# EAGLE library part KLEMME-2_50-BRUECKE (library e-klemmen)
Klemme 50-pol. mit Brückenhinweis
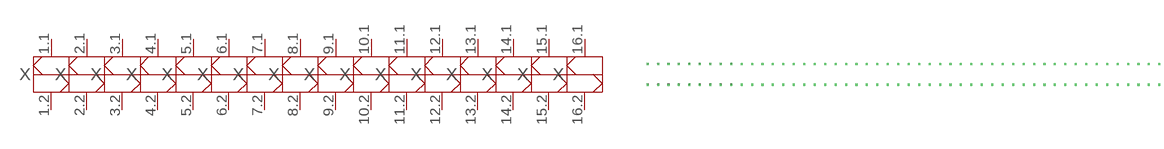
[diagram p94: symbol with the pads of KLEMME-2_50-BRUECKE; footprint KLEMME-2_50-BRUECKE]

Designator prefix X; gates 1=KLEMME-2_1-BRUECKE 2=KLEMME-2_2-BRUECKE 3=KLEMME-2_3-BRUECKE 4=KLEMME-2_4-BRUECKE 5=KLEMME-2_5-BRUECKE 6=KLEMME-2_6-BRUECKE 7=KLEMME-2_7-BRUECKE 8=KLEMME-2_8-BRUECKE 9=KLEMME-2_9-BRUECKE 10=KLEMME-2_10-BRUECKE 11=KLEMME-2_11-BRUECKE 12=KLEMME-2_12-BRUECKE 13=KLEMME-2_13-BRUECKE 14=KLEMME-2_14-BRUECKE 15=KLEMME-2_15-BRUECKE 16=KLEMME-2_16-BRUECKE 17=KLEMME-2_17-BRUECKE 18=KLEMME-2_18-BRUECKE 19=KLEMME-2_19-BRUECKE 20=KLEMME-2_20-BRUECKE 21=KLEMME-2_21-BRUECKE 22=KLEMME-2_22-BRUECKE 23=KLEMME-2_23-BRUECKE 24=KLEMME-2_24-BRUECKE 25=KLEMME-2_25-BRUECKE 26=KLEMME-2_26-BRUECKE 27=KLEMME-2_27-BRUECKE 28=KLEMME-2_28-BRUECKE 29=KLEMME-2_29-BRUECKE 30=KLEMME-2_30-BRUECKE 31=KLEMME-2_31-BRUECKE 32=KLEMME-2_32-BRUECKE 33=KLEMME-2_33-BRUECKE 34=KLEMME-2_34-BRUECKE 35=KLEMME-2_35-BRUECKE 36=KLEMME-2_36-BRUECKE 37=KLEMME-2_37-BRUECKE 38=KLEMME-2_38-BRUECKE 39=KLEMME-2_39-BRUECKE 40=KLEMME-2_40-BRUECKE 41=KLEMME-2_41-BRUECKE 42=KLEMME-2_42-BRUECKE 43=KLEMME-2_43-BRUECKE 44=KLEMME-2_44-BRUECKE 45=KLEMME-2_45-BRUECKE 46=KLEMME-2_46-BRUECKE 47=KLEMME-2_47-BRUECKE 48=KLEMME-2_48-BRUECKE 49=KLEMME-2_49-BRUECKE 50=KLEMME-2_50-BRUECKE

## KLEMME-2_50-BRUECKE  [KLEMME-2_50-BRUECKE]
1.1  1:1  pas
1.2  1:2  pas
2.1  2:1  pas
2.2  2:2  pas
3.1  3:1  pas
3.2  3:2  pas
4.1  4:1  pas
4.2  4:2  pas
5.1  5:1  pas
5.2  5:2  pas
6.1  6:1  pas
6.2  6:2  pas
7.1  7:1  pas
7.2  7:2  pas
8.1  8:1  pas
8.2  8:2  pas
9.1  9:1  pas
9.2  9:2  pas
10.1  10:1  pas
10.2  10:2  pas
11.1  11:1  pas
11.2  11:2  pas
12.1  12:1  pas
12.2  12:2  pas
13.1  13:1  pas
13.2  13:2  pas
14.1  14:1  pas
14.2  14:2  pas
15.1  15:1  pas
15.2  15:2  pas
16.1  16:1  pas
16.2  16:2  pas
17.1  17:1  pas
17.2  17:2  pas
18.1  18:1  pas
18.2  18:2  pas
19.1  19:1  pas
19.2  19:2  pas
20.1  20:1  pas
20.2  20:2  pas
21.1  21:1  pas
21.2  21:2  pas
22.1  22:1  pas
22.2  22:2  pas
23.1  23:1  pas
23.2  23:2  pas
24.1  24:1  pas
24.2  24:2  pas
25.1  25:1  pas
25.2  25:2  pas
26.1  26:1  pas
26.2  26:2  pas
27.1  27:1  pas
27.2  27:2  pas
28.1  28:1  pas
28.2  28:2  pas
29.1  29:1  pas
29.2  29:2  pas
30.1  30:1  pas
30.2  30:2  pas
31.1  31:1  pas
31.2  31:2  pas
32.1  32:1  pas
32.2  32:2  pas
33.1  33:1  pas
33.2  33:2  pas
34.1  34:1  pas
34.2  34:2  pas
35.1  35:1  pas
35.2  35:2  pas
36.1  36:1  pas
36.2  36:2  pas
37.1  37:1  pas
37.2  37:2  pas
38.1  38:1  pas
38.2  38:2  pas
39.1  39:1  pas
39.2  39:2  pas
40.1  40:1  pas
40.2  40:2  pas
41.1  41:1  pas
41.2  41:2  pas
42.1  42:1  pas
42.2  42:2  pas
43.1  43:1  pas
43.2  43:2  pas
44.1  44:1  pas
44.2  44:2  pas
45.1  45:1  pas
45.2  45:2  pas
46.1  46:1  pas
46.2  46:2  pas
47.1  47:1  pas
47.2  47:2  pas
48.1  48:1  pas
48.2  48:2  pas
49.1  49:1  pas
49.2  49:2  pas
50.1  50:1  pas
50.2  50:2  pas

## Footprint KLEMME-2_50-BRUECKE (pad centres in mm)
Dummy
drill 0.5 pad 1 square: 1.1 0,-2.54; 1.2 0,-12.7; 2.1 5.08,-2.54; 2.2 5.08,-12.7; 3.1 10.16,-2.54; 3.2 10.16,-12.7; 4.1 15.24,-2.54; 4.2 15.24,-12.7; 5.1 20.32,-2.54; 5.2 20.32,-12.7; 6.1 25.4,-2.54; 6.2 25.4,-12.7; 7.1 30.48,-2.54; 7.2 30.48,-12.7; 8.1 35.56,-2.54; 8.2 35.56,-12.7; 9.1 40.64,-2.54; 9.2 40.64,-12.7; 10.1 45.72,-2.54; 10.2 45.72,-12.7; 11.1 50.8,-2.54; 11.2 50.8,-12.7; 12.1 55.88,-2.54; 12.2 55.88,-12.7; 13.1 60.96,-2.54; 13.2 60.96,-12.7; 14.1 66.04,-2.54; 14.2 66.04,-12.7; 15.1 71.12,-2.54; 15.2 71.12,-12.7; 16.1 76.2,-2.54; 16.2 76.2,-12.7; 17.1 81.28,-2.54; 17.2 81.28,-12.7; 18.1 86.36,-2.54; 18.2 86.36,-12.7; 19.1 91.44,-2.54; 19.2 91.44,-12.7; 20.1 96.52,-2.54; 20.2 96.52,-12.7; 21.1 101.6,-2.54; 21.2 101.6,-12.7; 22.1 106.68,-2.54; 22.2 106.68,-12.7; 23.1 111.76,-2.54; 23.2 111.76,-12.7; 24.1 116.84,-2.54; 24.2 116.84,-12.7; 25.1 121.92,-2.54; 25.2 121.92,-12.7; 26.1 127,-2.54; 26.2 127,-12.7; 27.1 132.08,-2.54; 27.2 132.08,-12.7; 28.1 137.16,-2.54; 28.2 137.16,-12.7; 29.1 142.24,-2.54; 29.2 142.24,-12.7; 30.1 147.32,-2.54; 30.2 147.32,-12.7; 31.1 152.4,-2.54; 31.2 152.4,-12.7; 32.1 157.48,-2.54; 32.2 157.48,-12.7; 33.1 162.56,-2.54; 33.2 162.56,-12.7; 34.1 167.64,-2.54; 34.2 167.64,-12.7; 35.1 172.72,-2.54; 35.2 172.72,-12.7; 36.1 177.8,-2.54; 36.2 177.8,-12.7; 37.1 182.88,-2.54; 37.2 182.88,-12.7; 38.1 187.96,-2.54; 38.2 187.96,-12.7; 39.1 193.04,-2.54; 39.2 193.04,-12.7; 40.1 198.12,-2.54; 40.2 198.12,-12.7; 41.1 203.2,-2.54; 41.2 203.2,-12.7; 42.1 208.28,-2.54; 42.2 208.28,-12.7; 43.1 213.36,-2.54; 43.2 213.36,-12.7; 44.1 218.44,-2.54; 44.2 218.44,-12.7; 45.1 223.52,-2.54; 45.2 223.52,-12.7; 46.1 228.6,-2.54; 46.2 228.6,-12.7; 47.1 233.68,-2.54; 47.2 233.68,-12.7; 48.1 238.76,-2.54; 48.2 238.76,-12.7; 49.1 243.84,-2.54; 49.2 243.84,-12.7; 50.1 248.92,-2.54; 50.2 248.92,-12.7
